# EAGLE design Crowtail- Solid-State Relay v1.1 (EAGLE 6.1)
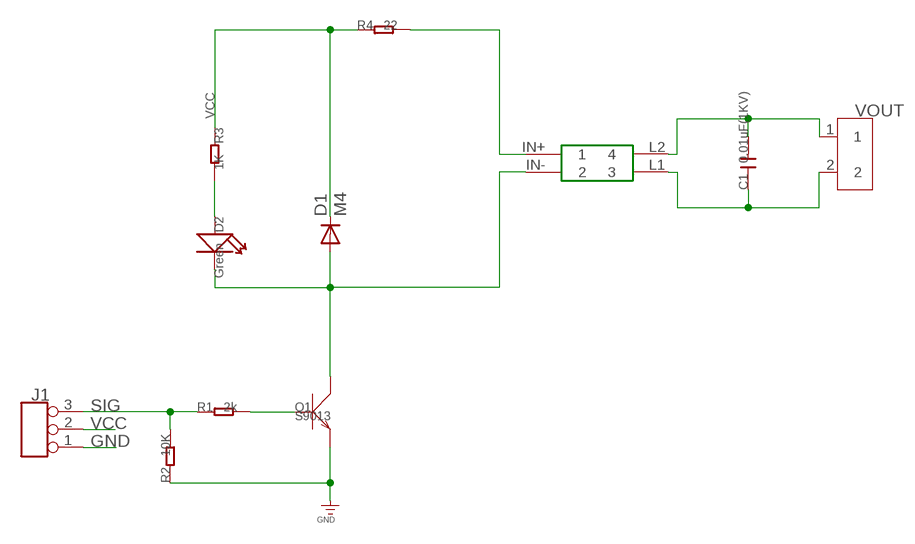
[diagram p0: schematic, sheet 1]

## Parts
C1  0.01uF(1KV)  C-1206  [C1206]
D1  M4  DIODE-DO-214AC  [DO-214AC]
D2  Green  LED'0603'  [LED-0603]
J1  TINKER_3P_DIP  [3P_2.0_DIP]
Q1  S9013  TRANSISTOR-NPN-SOT23  [SOT23]
R1  2k  R-0603  [R0603]
R2  10K  R-0603  [R0603]
R3  1K  R-0603  [R0603]
R4  22  R-0603  [R0603]
U$1  G3MB-202(RELAY)  [G3MB-202(RELAY)]
VOUT  SCREW-TERMINAL-2P'5.0'  [2P-5.0]

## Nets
GND: J1.1 Q1.2(E) R2.1
N$1: Q1.1(B) R1.2
N$2: D1.A D2.- Q1.3(C) U$1.IN-
N$3: R4.2 U$1.IN+
N$4: D2.+ R3.2
N$5: C1.2 U$1.L2 VOUT.1
N$6: C1.1 U$1.L1 VOUT.2
SIG: J1.3 R1.1 R2.2
VCC: D1.C J1.2 R3.1 R4.1

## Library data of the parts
C1 = Discrete:C*: Ceramic Capacitors
D1 = diode:DIODE-: DIODE
D2 = Discrete:LED*
J1 = Connector:TINKER_3P_DIP
Q1 = Discrete:TRANSISTOR-NPN*: NPN audion
R1-R4 = Discrete:R*
U$1 = G3MB-202(relay):G3MB-202(RELAY)
VOUT = Connector:SCREW-TERMINAL-2P

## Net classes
0 default: width 0.152 mm, drill 0.305 mm, clearance 0.152 mm
1 power: width 0.61 mm, drill 0.406 mm, clearance 0.203 mm
2 gnd: width 0.305 mm, drill 0.559 mm, clearance 0.254 mm
3 usbvcc: width 0.508 mm, drill 0.61 mm, clearance 0.254 mm

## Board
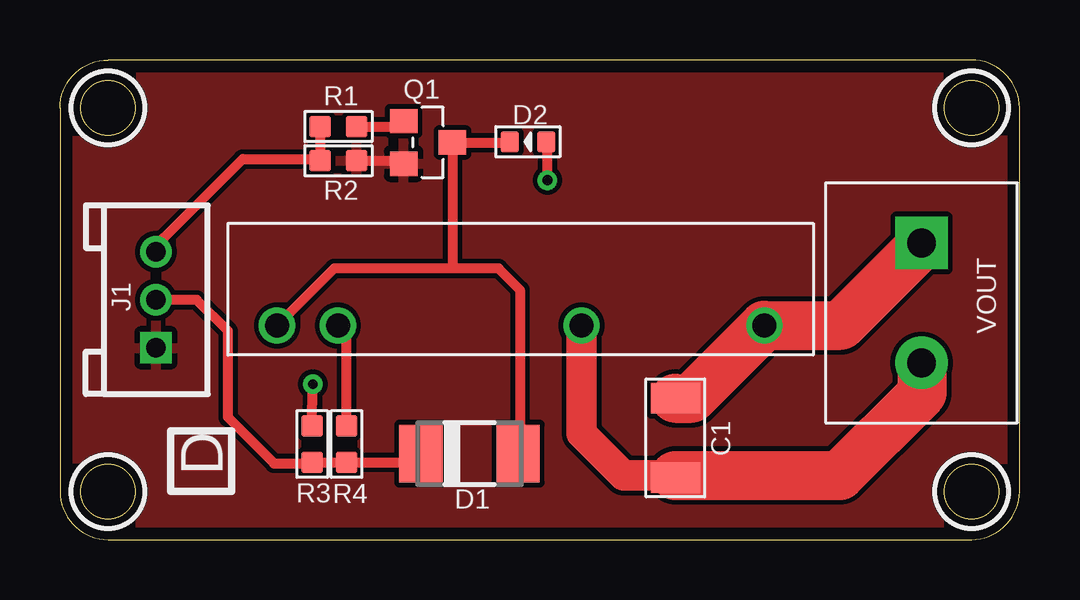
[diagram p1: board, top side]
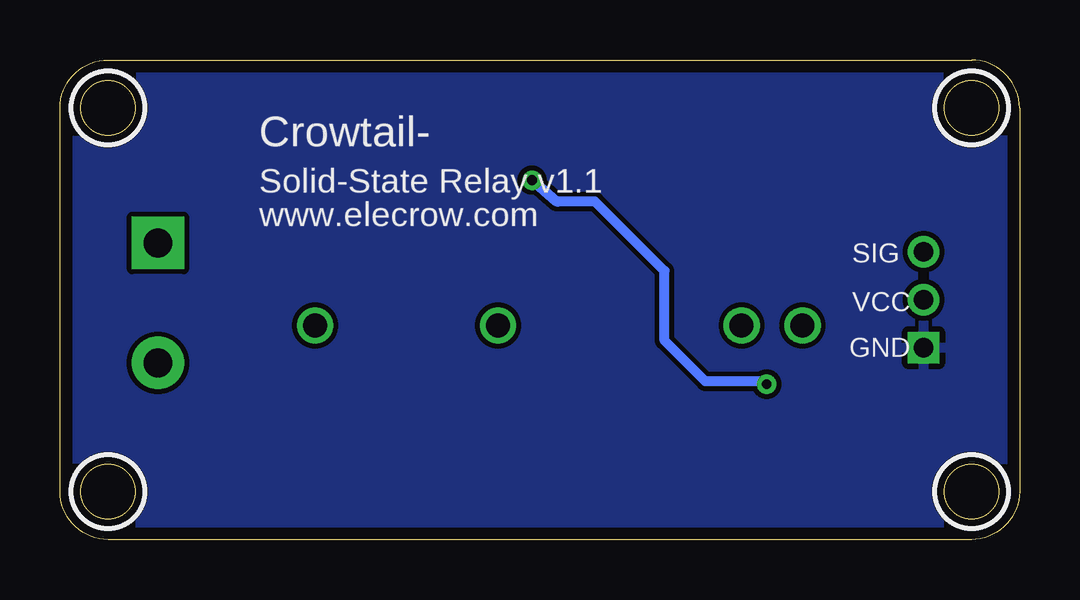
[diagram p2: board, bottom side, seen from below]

Size 40 x 20 mm. Coordinates in mm from the lower left corner, seen from the top.
Outline: 0,18 0,2 arc90 2,0 38,0 arc90 40,2 40,18 arc90 38,20 2,20 arc90 0,18
Outline: circle at 2,18 radius 1.14
Outline: circle at 2,2 radius 1.14
Outline: circle at 38,18 radius 1.14
Outline: circle at 38,2 radius 1.14
Copper layers (1*16): Top 0.035mm / dielectric 1.5mm / Bottom 0.035mm
Design rules: minimum track width 10mil, minimum drill 12mil, track to track 8mil, track to pad 8mil, pad to pad 8mil, via to via 8mil, smd to smd 10mil, copper to edge 20mil, drill to drill 8mil, minimum pad ring 10mil, minimum via ring 8mil, stop-mask expansion 2mil, vias tented up to drill 100mil, thermal gap 10mil
tRestrict: area 0.5,16.5 to 3.5,19.5; area 0.5,0.5 to 3.5,3.5; area 36.5,16.5 to 39.5,19.5; area 36.5,0.5 to 39.5,3.5
bRestrict: area 0.5,16.5 to 3.5,19.5; area 0.5,0.5 to 3.5,3.5; area 36.5,16.5 to 39.5,19.5; area 36.5,0.5 to 39.5,3.5

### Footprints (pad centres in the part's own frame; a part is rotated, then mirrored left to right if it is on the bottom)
C1206 = smd 1.27 x 2.032: 1 -1.651,0; 2 1.651,0
DO-214AC = smd 1.8 x 2.4: A 2.025,0; C -2.025,0
LED-0603 = smd 0.762 x 0.889: + -0.762,0; - 0.762,0
3P_2.0_DIP = drill 0.8 pad 1.27 square: 1 -2,0 | drill 0.8 pad 1.27: 2 0,0; 3 2,0
SOT23 = smd 1.016 x 1.143: 1 -0.889,-1.016; 2 0.889,-1.016; 3 0,1.016
R0603 = smd 0.889 x 0.889: 1 -0.762,0; 2 0.762,0
G3MB-202(RELAY) = drill 1: IN+ -7.62,2.54; IN- -10.16,2.54; L1 2.54,2.54; L2 10.16,2.54
2P-5.0 = drill 1.2 pad 2.184 square: 1 0,0 | drill 1.2 pad 2.184: 2 5,0

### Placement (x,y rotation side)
C1  25.65,4.24 90 top
D1  17.07,3.58 0 top
D2  19.51,16.59 180 top
J1  4,10 90 top
Q1  15.34,16.56 270 top
R1  11.61,17.22 0 top
R2  11.61,15.8 180 top
R3  10.52,3.99 90 top
R4  11.94,3.99 90 top
U$1  19.2,6.39 0 top
VOUT  35.92,12.37 270 top

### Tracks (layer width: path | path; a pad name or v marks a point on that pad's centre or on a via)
GND
  Top 0.406: R2.1 14.2,15.8 Q1.2
  pour Top: 0,20.32 40.64,20.32 40.64,0 0,0
  pour Bottom: 0,20.32 40.64,20.32 40.64,0 0,0
N$1
  Top 0.406: R1.2 14.17,17.22 14.35,17.4 14.35,17.42 Q1.1
N$2
  Top 0.406: D2.- 18.72,16.56 Q1.3 16.36,11.4 16.26,11.3 | 16.26,11.3 18.29,11.3 19.18,10.41 19.18,3.56 | 16.26,11.3 11.43,11.3 9.02,8.89 9.02,8.9 U$1.IN- | 19.18,3.56 19.05,3.43 | 19.18,3.56 19.12,3.56 D1.A
N$3
  Top 0.406: R4.2 11.94,8.56 11.58,8.92 U$1.IN+
N$4  (via drill 0.41)
  Top 0.406: R3.2 v10.54,6.48 | v20.32,14.99 20.32,16.54 D2.+
  Bottom 0.406: v10.54,6.48 10.54,6.6 13.1,6.6 14.8,8.3 14.8,11.2 17.7,14.1 19.2,14.1 19.3,14.1 v20.32,14.99
N$5
  Top 2.032: C1.2 26.32,5.89 U$1.L2 32.55,8.93 35.81,12.19 35.81,12.32 35.92,12.42 | VOUT.1 35.92,12.42 | 35.92,12.42 35.94,12.45
N$6
  Top 1.016: C1.1 25.65,2.67
  Top 1.27: U$1.L1 21.74,4.42 23.5,2.67 25.58,2.67 C1.1
  Top 2.032: 25.65,2.67 32.51,2.67 35.94,6.1 35.94,7.37 VOUT.2
SIG
  Top 0.406: R1.1 R2.2 10.77,15.88 7.62,15.88 4.32,12.57 J1.3
VCC
  Top 0.406: J1.2 5.7,10 7,8.7 7,5.1 8.93,3.17 10.46,3.17 R3.1 R4.1 14.69,3.23 D1.C

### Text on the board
tPlace: D
bPlace: Crowtail- | Solid-State Relay v1.1 | www.elecrow.com | SIG | VCC | GND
